FUNCTION_BLOCK FB 138
TITLE =TRASFERIMENTO PARAMETRI AZIONAMENTO 8 NASTRI
VERSION : 0.1

BEGIN
NETWORK
TITLE =START SCRITTURA PARAMETRO 1 SE VIENE VARIATO PKE/INDEX/VALORE
//D12 VELOCITA BASSA=VELOCITA' LINEA
//
//      L     DB100.DBD  132              //VELOCITA LINEA' =J10 MASTER
//      T     DB100.DBD  800


      L     DB100.DBD  800;
      L     DB108.DBD  100;
      ==D   ;
      SPB   _006;

      L     1060;
      T     DB108.DBW   20;
      L     12;
      T     DB108.DBW   22;
      L     DB100.DBD  800;
      T     DB108.DBD   24;
      =     M     26.0;
_006: NOP   0;

NETWORK
TITLE =START SCRITTURA PARAMETRO 2 SE VIENE VARIATO PKE/INDEX/VALORE
//D22 VELOCITA' ALTA
      L     DB100.DBD  804;
      L     DB108.DBD  104;
      ==D   ;
      SPB   _007;

      L     1060;
      T     DB108.DBW   20;

      L     22;
      T     DB108.DBW   22;

      L     DB100.DBD  804;
      T     DB108.DBD   24;
      =     M     26.1;
_007: NOP   0;

NETWORK
TITLE =START SCRITTURA PARAMETRO 3 SE VIENE VARIATO PKE/INDEX/VALORE
//D10 ACCELERAZIONE LENTA
      L     DB100.DBD  808;
      L     DB108.DBD  108;
      ==D   ;
      SPB   _008;

      L     1060;
      T     DB108.DBW   20;
      L     10;
      T     DB108.DBW   22;
      L     DB100.DBD  808;
      T     DB108.DBD   24;
      =     M     26.2;
      SPA   _009;
_008: NOP   0;

NETWORK
TITLE =START SCRITTURA PARAMETRO 4 SE VIENE VARIATO PKE/INDEX/VALORE
//D20 ACCELERAZIONE VELOCE
      L     DB100.DBD  808;
      T     DB100.DBD  812;

      L     DB100.DBD  812;
      L     DB108.DBD  112;
      ==D   ;
      SPB   _009;

      L     1060;
      T     DB108.DBW   20;
      L     20;
      T     DB108.DBW   22;
      L     DB100.DBD  812;
      T     DB108.DBD   24;
      =     M     26.3;
_009: NOP   0;

NETWORK
TITLE =START SCRITTURA PARAMETRO 5 SE VIENE VARIATO PKE/INDEX/VALORE
//D11 DECELERAZIONE LENTA
//
      L     DB100.DBD  816;
      L     DB108.DBD  116;
      ==D   ;
      SPB   _010;

      L     1060;
      T     DB108.DBW   20;
      L     11;
      T     DB108.DBW   22;
      L     DB100.DBD  816;
      T     DB108.DBD   24;
      =     M     26.4;
      SPA   _011;
_010: NOP   0;

NETWORK
TITLE =START SCRITTURA PARAMETRO 6 SE VIENE VARIATO PKE/INDEX/VALORE
//D21 DECELERAZIONE VELOCE
      L     DB100.DBD  816;
      T     DB100.DBD  820;

      L     DB100.DBD  820;
      L     DB108.DBD  120;
      ==D   ;
      SPB   _011;

      L     1060;
      T     DB108.DBW   20;
      L     21;
      T     DB108.DBW   22;
      L     DB100.DBD  820;
      T     DB108.DBD   24;
      =     M     26.5;
_011: NOP   0;

NETWORK
TITLE =START SCRITTURA PARAMETRO 7 SE VIENE VARIATO PKE/INDEX/VALORE

      L     DB100.DBD  824;
      L     DB108.DBD  124;
      ==D   ;
      SPB   _012;

      L     1160;
      T     DB108.DBW   20;
      L     21;
      T     DB108.DBW   22;
      L     DB100.DBD  824;
      T     DB108.DBD   24;
//    =     M     26.6
_012: NOP   0;

NETWORK
TITLE =START SCRITTURA PARAMETRO 8 SE VIENE VARIATO PKE/INDEX/VALORE
//
//

      L     DB100.DBD  828;
      L     DB108.DBD  128;
      ==D   ;

      SPB   _013;
      L     1060;
      T     DB108.DBW   20;
      L     22;
      T     DB108.DBW   22;
      L     DB100.DBD  828;
      T     DB108.DBD   24;
//      =     M     26.7
_013: NOP   0;

NETWORK
TITLE =START SCRITTURA PARAMETRO 9 SE VIENE VARIATO PKE/INDEX/VALORE
//VELOCITA' BASSA=VALOCITA' LINEA

      L     DB100.DBD  832;
      L     DB108.DBD  132;
      ==D   ;
      SPB   _014;

      L     1060;
      T     DB108.DBW   20;
      L     12;
      T     DB108.DBW   22;
      L     DB100.DBD  832;
      T     DB108.DBD   24;
//   =     M     27.0
_014: NOP   0;

NETWORK
TITLE =START SCRITTURA PARAMETRO 10 SE VIENE VARIATO PKE/INDEX/VALORE

      L     DB100.DBD  836;
      L     DB108.DBD  136;
      ==D   ;
      SPB   _015;
      L     1180;
      T     DB108.DBW   20;
      L     30;
      T     DB108.DBW   22;
      L     DB100.DBD  836;
      T     DB108.DBD   24;
//    =     M     27.1
_015: NOP   0;

NETWORK
TITLE =START SCRITTURA PARAMETRO 11 SE VIENE VARIATO PKE/INDEX/VALORE

      L     DB100.DBD  840;
      L     DB108.DBD  140;
      ==D   ;
      SPB   _016;
      L     1180;
      T     DB108.DBW   20;
      L     30;
      T     DB108.DBW   22;
      L     DB100.DBD  840;
      T     DB108.DBD   24;
//    =     M     27.2
_016: NOP   0;

NETWORK
TITLE =START SCRITTURA PARAMETRO 12 SE VIENE VARIATO PKE/INDEX/VALORE

      L     DB100.DBD  844;
      L     DB108.DBD  144;
      ==D   ;
      SPB   _017;
      L     1180;
      T     DB108.DBW   20;
      L     30;
      T     DB108.DBW   22;
      L     DB100.DBD  844;
      T     DB108.DBD   24;
//   =     M     27.3
_017: NOP   0;

NETWORK
TITLE =START SCRITTURA PARAMETRO 13 SE VIENE VARIATO PKE/INDEX/VALORE

      L     DB100.DBD  848;
      L     DB108.DBD  148;
      ==D   ;
      SPB   _018;
      L     1180;
      T     DB108.DBW   20;
      L     30;
      T     DB108.DBW   22;
      L     DB108.DBD  848;
      T     DB108.DBD   24;
//   =     M     27.4
_018: NOP   0;

NETWORK
TITLE =START SCRITTURA PARAMETRO 14 SE VIENE VARIATO PKE/INDEX/VALORE

      L     DB100.DBD  852;
      L     DB108.DBD  152;
      ==D   ;
      SPB   _019;
      L     1180;
      T     DB108.DBW   20;
      L     30;
      T     DB108.DBW   22;
      L     DB100.DBD  852;
      T     DB108.DBD   24;
//     =     M     27.5
_019: NOP   0;

NETWORK
TITLE =START SCRITTURA PARAMETRO 15 SE VIENE VARIATO PKE/INDEX/VALORE

      L     DB100.DBD  856;
      L     DB108.DBD  156;
      ==D   ;
      SPB   _020;

      L     1180;
      T     DB108.DBW   20;
      L     30;
      T     DB108.DBW   22;
      L     DB100.DBD  856;
      T     DB108.DBD   24;
//    =     M     27.6
_020: NOP   0;

NETWORK
TITLE =START SCRITTURA PARAMETRO 16 SE VIENE VARIATO PKE/INDEX/VALORE

      L     DB100.DBD  860;
      L     DB108.DBD  160;
      ==D   ;
      SPB   _021;
      L     1180;
      T     DB108.DBW   20;
      L     30;
      T     DB108.DBW   22;
      L     DB100.DBD  860;
      T     DB108.DBD   24;
//     =     M     27.7
_021: NOP   0;

NETWORK
TITLE =START SCRITTURA PARAMETRO 17 SE VIENE VARIATO PKE/INDEX/VALORE

      L     DB100.DBD  864;
      L     DB108.DBD  164;
      ==D   ;
      SPB   _022;
      L     1180;
      T     DB108.DBW   20;
      L     30;
      T     DB108.DBW   22;
      L     DB100.DBD  864;
      T     DB108.DBD   24;
//     =     M     28.0
_022: NOP   0;

NETWORK
TITLE =START SCRITTURA PARAMETRO 18 SE VIENE VARIATO PKE/INDEX/VALORE

      L     DB100.DBD  868;
      L     DB108.DBD  168;
      ==D   ;
      SPB   _023;
      L     1180;
      T     DB108.DBW   20;
      L     30;
      T     DB108.DBW   22;
      L     DB100.DBD  868;
      T     DB108.DBD   24;
//     =     M     28.1
_023: NOP   0;

NETWORK
TITLE =START SCRITTURA PARAMETRO 19 SE VIENE VARIATO PKE/INDEX/VALORE

      L     DB100.DBD  872;
      L     DB108.DBD  172;
      ==D   ;
      SPB   _024;
      L     1180;
      T     DB108.DBW   20;
      L     30;
      T     DB108.DBW   22;
      L     DB100.DBD  872;
      T     DB108.DBD   24;
//     =     M     28.2
_024: NOP   0;

NETWORK
TITLE =START SCRITTURA PARAMETRO 20 SE VIENE VARIATO PKE/INDEX/VALORE

      L     DB100.DBD  876;
      L     DB108.DBD  176;
      ==D   ;
      SPB   _025;
      L     1180;
      T     DB108.DBW   20;
      L     30;
      T     DB108.DBW   22;
      L     DB100.DBD  876;
      T     DB108.DBD   24;
//     =     M     28.3
_025: NOP   0;

NETWORK
TITLE =START SCRITTURA PARAMETRI
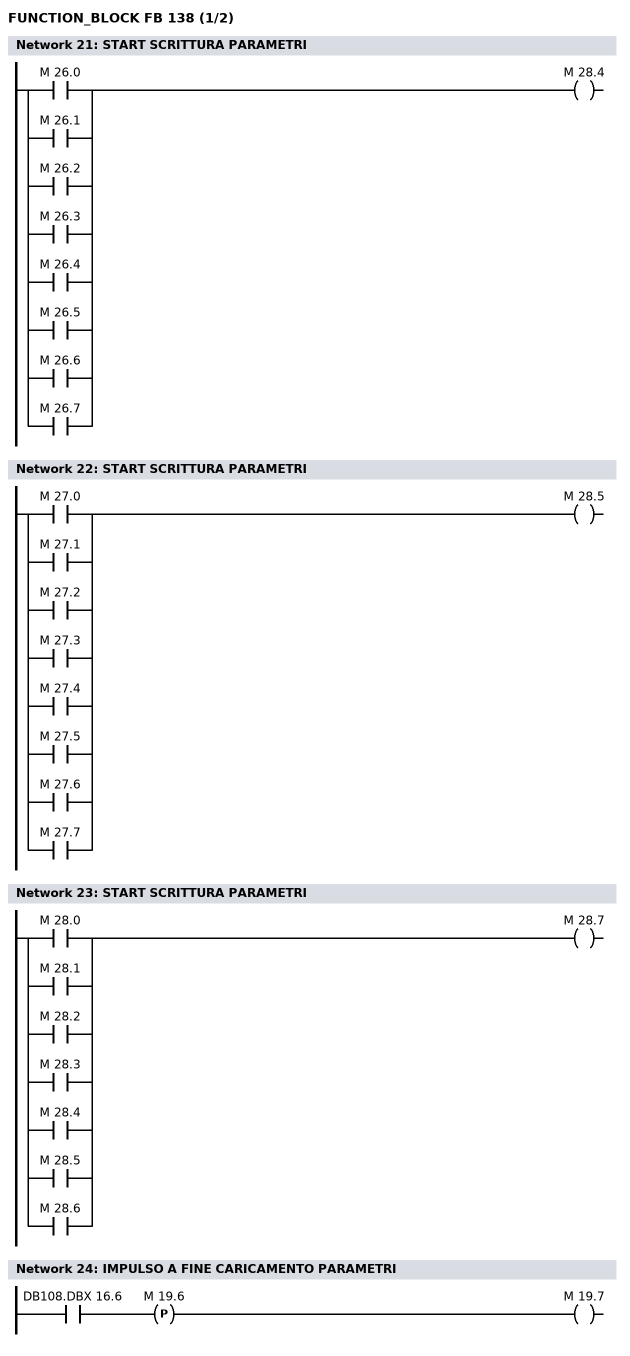
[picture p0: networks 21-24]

      O     M     26.0;
      O     M     26.1;
      O     M     26.2;
      O     M     26.3;
      O     M     26.4;
      O     M     26.5;
      O     M     26.6;
      O     M     26.7;
      =     M     28.4;
NETWORK
TITLE =START SCRITTURA PARAMETRI

      O     M     27.0;
      O     M     27.1;
      O     M     27.2;
      O     M     27.3;
      O     M     27.4;
      O     M     27.5;
      O     M     27.6;
      O     M     27.7;
      =     M     28.5;
NETWORK
TITLE =START SCRITTURA PARAMETRI

      O     M     28.0;
      O     M     28.1;
      O     M     28.2;
      O     M     28.3;
      O     M     28.4;
      O     M     28.5;
      O     M     28.6;
      =     M     28.7;
NETWORK
TITLE =IMPULSO A FINE CARICAMENTO PARAMETRI

      U     DB108.DBX   16.6;
      FP    M     19.6;
      =     M     19.7;
NETWORK
TITLE =START SALVATAGGIO PARAMETRI A FINE CARICAMENTO VALORI
//TOGLIENO M280.0 OGNI VOLTA CHE VIENE CAMBIATO UN VALORE ESEGUI A00=SALVA
//PARAMETRI
//
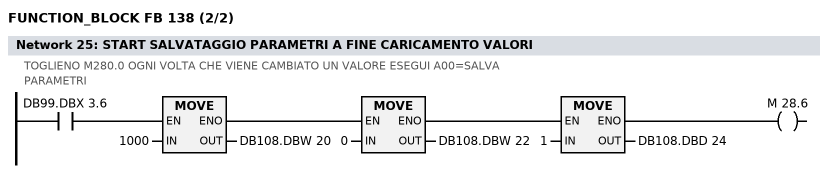
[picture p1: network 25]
      U(    ;
      U(    ;
      U     DB99.DBX    3.6;
      SPBNB _001;
      L     1000;
      T     DB108.DBW   20;
      SET   ;
      SAVE  ;
      CLR   ;
_001: U     BIE;
      )     ;
      SPBNB _002;
      L     0;
      T     DB108.DBW   22;
      SET   ;
      SAVE  ;
      CLR   ;
_002: U     BIE;
      )     ;
      SPBNB _003;
      L     1;
      T     DB108.DBD   24;
      SET   ;
      SAVE  ;
      CLR   ;
_003: U     BIE;
      =     M     28.6;
NETWORK
TITLE =VALORE DI RITORNO A COMANDO ACCETTATO

      UN    M     19.7;

      SPB   _030;
      L     DB100.DBD  800;
      T     DB108.DBD  100;
      R     M     26.0;

      L     DB100.DBD  804;
      T     DB108.DBD  104;
      R     M     26.1;

      L     DB100.DBD  808;
      T     DB108.DBD  108;
      R     M     26.2;

      L     DB100.DBD  812;
      T     DB108.DBD  112;
      R     M     26.3;

      L     DB100.DBD  816;
      T     DB108.DBD  116;
      R     M     26.4;

      L     DB100.DBD  820;
      T     DB108.DBD  120;
      R     M     26.5;

      L     DB100.DBD  824;
      T     DB108.DBD  124;
      R     M     26.6;

      L     DB100.DBD  828;
      T     DB108.DBD  128;
      R     M     26.7;

      L     DB100.DBD  832;
      T     DB108.DBD  132;
      R     M     27.0;

      L     DB100.DBD  836;
      T     DB108.DBD  136;
      R     M     27.1;

      L     DB100.DBD  840;
      T     DB108.DBD  140;
      R     M     27.2;

      L     DB100.DBD  844;
      T     DB108.DBD  144;
      R     M     27.3;

      L     DB100.DBD  848;
      T     DB108.DBD  148;
      R     M     27.4;

      L     DB100.DBD  852;
      T     DB108.DBD  152;
      R     M     27.5;

      L     DB100.DBD  856;
      T     DB108.DBD  156;
      R     M     27.6;

      L     DB100.DBD  860;
      T     DB108.DBD  160;
      R     M     27.7;

      L     DB100.DBD  864;
      T     DB108.DBD  164;
      R     M     28.0;

      L     DB100.DBD  868;
      T     DB108.DBD  168;
      R     M     28.1;

      L     DB100.DBD  872;
      T     DB108.DBD  172;
      R     M     28.2;

      L     DB100.DBD  876;
      T     DB108.DBD  176;
      R     M     28.3;

_030: NOP   0;

NETWORK
TITLE =

      U     DB108.DBX   16.4; // START SCRITTURA DATI
      SPB   M001;
      L     0;
      T     DB108.DBW    8; // AZZERAMENTO PKE
      CALL "DPWR_DAT" (
           LADDR                    := W#16#154,
           RECORD                   := P#DB108.DBX 8.0 BYTE 8,
           RET_VAL                  := DB108.DBW   30);

M001: U     M     28.7; // ABILITA SCRITTURA DATI

      UN    DB108.DBX   16.4;
      S     DB108.DBX   16.4;
      R     DB108.DBX   16.5;
      R     DB108.DBX   16.6;
      UN    DB108.DBX   16.4;
      SPB   M002;

// TRASFERISCO NUMERO DEL PARAMETRO (PKE)


      L     DB108.DBW   20; // PKE  VEDI MANUALE PROFIBUS
      T     DB108.DBW    8;
      U     DB108.DBX   16.4;
      R     DB108.DBX    8.3;
      S     DB108.DBX    8.4; // LANCIO JOB SCRITTURA DATI MANUALE PROF.PAG.7
      S     DB108.DBX    8.5;
      R     DB108.DBX    8.6;

// NUOVO INDEX

      L     DB108.DBW   22; // INDEX VEDI MANUALE PROFIBUS
      TAW   ;
      T     DB108.DBW   10;

// VALORE DA TRASFERIRE

      L     DB108.DBD   24; // VALORE DA TRASFERIRE
      T     DB108.DBD   12;

// LANCIO LA SCRITTURA DEI DATI

      CALL "DPWR_DAT" (
           LADDR                    := W#16#154,
           RECORD                   := P#DB108.DBX 8.0 BYTE 8,
           RET_VAL                  := DB108.DBW   32);
      SET   ;
      R     DB108.DBX   16.4;
      S     DB108.DBX   16.5; // FINE DELLA SCRITTURA DATI

// RITORNO DEI DATI TRASMESSI

      CALL "DPRD_DAT" (
           LADDR                    := W#16#154,
           RET_VAL                  := DB108.DBW   34,
           RECORD                   := P#DB108.DBX 8.0 BYTE 8);
      UN    DB108.DBX    8.4;
      U     DB108.DBX    8.5;
      UN    DB108.DBX    8.6;
      S     DB108.DBX   16.6; // DATI CORRETTAMENTE INSERITI

M002: NOP   1;

END_FUNCTION_BLOCK

